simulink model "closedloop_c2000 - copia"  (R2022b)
settings: Solver=VariableStepAuto  StartTime=0.0  StopTime=10.0  RelTol=1e-3
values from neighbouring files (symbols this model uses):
  kaw = ki/kp    (= 100)    [closedloop_analysis - copia.m]
  ki = wc*R    (= 20)    [closedloop_analysis - copia.m]
  kp = wc*L    (= 0.2)    [closedloop_analysis - copia.m]
  PWMcounter_period = floor(fcpu/fsw)    [closedloop_analysis - copia.m]
  Ts = Tsw    (= 2.77777777778e-05)    [closedloop_analysis - copia.m]
  Vdc = 450    [closedloop_analysis - copia.m]
undefined symbols (not defined in the file or in its folder): ADCIN0, ADCIN1, ADCINA0, ADCINB0, bit, DCAEVT1, DCAEVT1FILT, Down, ended, Filtered, g_adc, input, of, offset, Single, Trip, TZ1, Up, version, Zone
libraries: c2802xlib x7, simulink x2, slpidlib x2

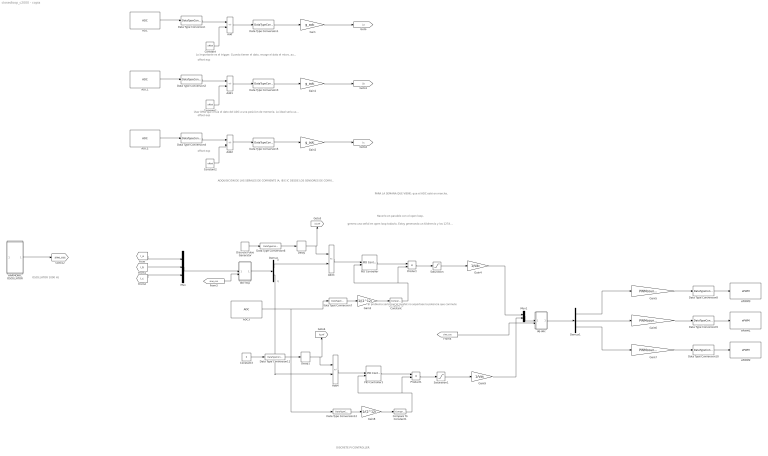
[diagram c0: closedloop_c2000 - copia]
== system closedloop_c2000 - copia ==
  note: PARA LA SEMANA QUE VIENE: que el ADC esté en marcha.
  note: El problema sería que el mosfet no soportase la potencia que conmute
  note: genero una señal en open loop todavía. Estoy generando un kilohercio y los 127A de pico. En teoría, el bucle cerrado tiene que estar midienddo esas dos partes de error, 0 prácticamente. Debería comportarse como el open loop. En el momento en el que cambias las consignas de bucle cerrado, el va a intentar modificar los PWMs porque le va a estar dando error. Ahí los PI se ponen en marchas y generan diferencias en las consignas de salida, y como la inyección siguie siendo del open loop, se van a saturar los PI porque por mucho que intenta el control llevar la señal, como las señales serán fijas, no hay modificación, el error se aculuma y se saturará.
  note: Hacerlo en paralelo con el open loop.
  note: Usar DMA que envia el dato del ADC a una posicion de memoria. Lo ideal seria usarlo. Avisa a un elemento y lo pone en posiciopn X. cuando lanza la interrupcion de procesado. Le podemos decir que solo avise al micro solo cuando los ADCs hayan terminado. Tenemos está opcion. Si no es grave el desfase, se puede dejar así, si vemos que necesitamos más precisión, mejor.
  note: Lo importante es el trigger. Cuando tienen el dato, recoge el dato el micro, aunque no sea en el mismo instante temporal, el tiempo de retardo debería ser despreciable.
  note: OSCILLATOR 1000 Hz
  note: DISCRETE PI CONTROLLER
  note: q
  note: d
  note: ADQUISICIÓN DE LAS SEÑALES DE CORRIENTE IA, IB E IC DESDE LOS SENSORES DE CORRIENTE HASTA EL MICRO A TRAVÉS DE LOS ADC
  note: offset exp
  note: offset exp
  note: offset exp
  ADC : c2802xlib/ADC  blkParamProc=C2000  ADCModule=1  samplingMode=Single sample mode  ADCResolution=12-bit (Single-ended input)  useSOC1=SOC0  useSOC2=SOC0_SOC1  SOCAcquisitionWindow=7  SOCTriggerSource=ePWM1_ADCSOCA  SOCInterruptTrigger=No ADCINT  Ts=Ts  dType=uint16  postInterrupt=off  interruptSel=ADCINT1  ADCINTContinuous=on  endma=off  chdma=1  conv1=ADCINA0  conv2=ADCINA0 and ADCINB0  conv1_Type4=ADCIN0  conv2_Type4=ADCIN0 and ADCIN1
  ADC1 : c2802xlib/ADC  blkParamProc=C2000  ADCModule=1  samplingMode=Single sample mode  ADCResolution=12-bit (Single-ended input)  useSOC1=SOC1  useSOC2=SOC0_SOC1  SOCAcquisitionWindow=7  SOCTriggerSource=ePWM1_ADCSOCA  SOCInterruptTrigger=No ADCINT  Ts=Ts  dType=uint16  postInterrupt=off  interruptSel=ADCINT1  ADCINTContinuous=off  endma=off  chdma=1  conv1=ADCINA1  conv2=ADCINA0 and ADCINB0  conv1_Type4=ADCIN0  conv2_Type4=ADCIN0 and ADCIN1
  ADC2 : c2802xlib/ADC  blkParamProc=C2000  ADCModule=1  samplingMode=Single sample mode  ADCResolution=12-bit (Single-ended input)  useSOC1=SOC3  useSOC2=SOC0_SOC1  SOCAcquisitionWindow=7  SOCTriggerSource=ePWM1_ADCSOCA  SOCInterruptTrigger=No ADCINT  Ts=Ts  dType=uint16  postInterrupt=off  interruptSel=ADCINT1  ADCINTContinuous=off  endma=off  chdma=1  conv1=ADCINA2  conv2=ADCINA0 and ADCINB0  conv1_Type4=ADCIN0  conv2_Type4=ADCIN0 and ADCIN1
  ADC3 : c2802xlib/ADC  blkParamProc=C2000  ADCModule=1  samplingMode=Single sample mode  ADCResolution=12-bit (Single-ended input)  useSOC1=SOC0  useSOC2=SOC0_SOC1  SOCAcquisitionWindow=7  SOCTriggerSource=Software  SOCInterruptTrigger=No ADCINT  Ts=0.0011  dType=uint16  postInterrupt=off  interruptSel=ADCINT1  ADCINTContinuous=off  endma=off  chdma=1  conv1=ADCINB3  conv2=ADCINA0 and ADCINB0  conv1_Type4=ADCIN0  conv2_Type4=ADCIN0 and ADCIN1
  Add{,1..4} (5 alike) : Sum  Inputs=+-
  Compare To Constant : simulink/Logic and Bit Operations/Compare To Constant  relop=>=  const=0.5  OutDataTypeStr=boolean
  Compare To Constant1 : simulink/Logic and Bit Operations/Compare To Constant  relop=>=  const=0.5  OutDataTypeStr=boolean
  Constant : Constant  Value=offset
  Constant1 : Constant  Value=offset
  Constant2 : Constant  Value=offset
  Constant3 : Constant  Value=0
  Data Type Conversion{,2,4,7..10,12} (8 alike) : DataTypeConversion  OutDataTypeStr=int16
  Data Type Conversion{1,3,5..6,11} (5 alike) : DataTypeConversion  OutDataTypeStr=single
  Delay : Delay  DelayLength=1  SampleTime=Ts/2
  Delay1 : Delay  DelayLength=1  SampleTime=Ts/2
  Demux : Demux  Outputs=2
  Demux1 : Demux  Outputs=3
  Discrete Pulse Generator : DiscretePulseGenerator  Amplitude=127  Period=120  PulseWidth=60  PhaseDelay=5  SampleTime=Ts
  Gain : Gain  Gain=g_adc
  Gain1 : Gain  Gain=g_adc
  Gain2 : Gain  Gain=g_adc
  Gain3 : Gain  Gain=1/(2^12)
  Gain4 : Gain  Gain=1/Vdc
  Gain5 : Gain  Gain=PWMcounter_period
  Gain6 : Gain  Gain=PWMcounter_period
  Gain7 : Gain  Gain=PWMcounter_period
  Gain8 : Gain  Gain=1/(2^12)
  Gain9 : Gain  Gain=1/Vdc
  HARMONIC OSCILLATOR : Subsystem
  Mux : Mux  Inputs=3
  Mux1 : Mux  Inputs=2
  PID Controller : slpidlib/PID Controller  Controller=PI  Form=Parallel  TimeDomain=Discrete-time  UseExternalTs=off  SampleTime=Ts  IntegratorMethod=Backward Euler  FilterMethod=Forward Euler  ControllerParametersSource=internal  P=kp  I=ki  UseKiTs=off  D=0  N=100  UseFilter=on  TunerSelectOption=Frequency Response Based  InitialConditionSource=internal  InitialConditionForIntegrator=0  InitialConditionForFilter=0  DifferentiatorICPrevScaledInput=0  ExternalReset=rising  TrackingMode=off  Kt=1  LimitOutput=on  SatLimitsSource=internal  UpperSaturationLimit=Vdc*0.98  LowerSaturationLimit=0  LinearizeAsGain=on  AntiWindupMode=back-calculation  Kb=kaw  LimitIntegrator=off  UpperIntegratorSaturationLimit=inf  LowerIntegratorSaturationLimit=-inf  POutMin=[]  POutMax=[]  IOutMin=[]  IOutMax=[]  DOutMin=[]  DOutMax=[]  NOutMin=[]  NOutMax=[]  SumOutMin=[]  SumOutMax=[]  SaturationOutMin=[]  SaturationOutMax=[]  PParamMin=[]  PParamMax=[]  IParamMin=[]  IParamMax=[]  DParamMin=[]  DParamMax=[]  NParamMin=[]  NParamMax=[]  KbParamMin=[]  KbParamMax=[]  KtParamMin=[]  KtParamMax=[]  KbOutMin=[]  KbOutMax=[]  KtOutMin=[]  KtOutMax=[]  IntegratorOutMin=[]  IntegratorOutMax=[]  FilterOutMin=[]  FilterOutMax=[]  SumI1OutMin=[]  SumI1OutMax=[]  SumI2OutMin=[]  SumI2OutMax=[]  SumI3OutMin=[]  SumI3OutMax=[]  SumI4OutMin=[]  SumI4OutMax=[]  SumDOutMin=[]  SumDOutMax=[]  DifferentiatorOutMin=[]  DifferentiatorOutMax=[]  FilterDiffOutCoefMin=[]  FilterDiffOutCoefMax=[]  ReciprocalOutMin=[]  ReciprocalOutMax=[]  SumDenOutMin=[]  SumDenOutMax=[]  SumNumOutMin=[]  SumNumOutMax=[]  DivideOutMin=[]  DivideOutMax=[]  UdiffTsProdOutMin=[]  UdiffTsProdOutMax=[]  NTsProdOutMin=[]  NTsProdOutMax=[]  UintegralTsProdOutMin=[]  UintegralTsProdOutMax=[]  UngainTsProdOutMin=[]  UngainTsProdOutMax=[]  ClampingZeroOutDataTypeStr=Inherit: Inherit via back propagation  ClampingZeroOutMin=[]  ClampingZeroOutMax=[]  FilterDenConstantOutDataTypeStr=Inherit: Inherit via back propagation  FilterDenConstantOutMin=[]  FilterDenConstantOutMax=[]  PCopyOutDataTypeStr=Inherit: Inherit via back propagation  PCopyOutMin=[]  PCopyOutMax=[]  NCopyOutDataTypeStr=Inherit: Inherit via back propagation  NCopyOutMin=[]  NCopyOutMax=[]  IntegratorContinuousStateAttributes=''  IntegratorStateMustResolveToSignalObject=off  IntegratorRTWStateStorageClass=Auto  FilterContinuousStateAttributes=''  FilterStateMustResolveToSignalObject=off  FilterRTWStateStorageClass=Auto  ParallelPVariant=InternalParameters  IdealPVariant=Disabled  IVariant=InternalParameters  DVariant=Disabled  IntegratorVariant=Discrete  SatVariant=Enabled  AWVariant=BackCalculation  PCopyVariant=Disabled  TRVariant=Disabled  FdbkBlocksVariant=Feedback  IdealPFdbkVariant=Passthrough  SatFdbkVariant=Enabled  DerivativeFilterVariant=Disabled  NVariant=Disabled  NCopyVariant=Disabled_SignalSpec  FilterICVariant=Disabled  IntegratorICVariant=InternalICs  ExternalResetVariant=ExternalReset  TRSumVariant=Passthrough  SumFdbkVariant=Enabled  SumVariant=Sum_PI  TsampFilterVariant=InternalTs  TsampNgainVariant=Passthrough  TsampIntegralVariant=Passthrough  ExternalSaturationOutDataTypeStr=Inherit: Same as second input
  PID Controller1 : slpidlib/PID Controller  Controller=PI  Form=Parallel  TimeDomain=Discrete-time  UseExternalTs=off  SampleTime=Ts  IntegratorMethod=Backward Euler  FilterMethod=Forward Euler  ControllerParametersSource=internal  P=kp  I=ki  UseKiTs=off  D=0  N=100  UseFilter=on  TunerSelectOption=Frequency Response Based  InitialConditionSource=internal  InitialConditionForIntegrator=0  InitialConditionForFilter=0  DifferentiatorICPrevScaledInput=0  ExternalReset=rising  TrackingMode=off  Kt=1  LimitOutput=on  SatLimitsSource=internal  UpperSaturationLimit=Vdc*0.98  LowerSaturationLimit=0  LinearizeAsGain=on  AntiWindupMode=back-calculation  Kb=kaw  LimitIntegrator=off  UpperIntegratorSaturationLimit=inf  LowerIntegratorSaturationLimit=-inf  POutMin=[]  POutMax=[]  IOutMin=[]  IOutMax=[]  DOutMin=[]  DOutMax=[]  NOutMin=[]  NOutMax=[]  SumOutMin=[]  SumOutMax=[]  SaturationOutMin=[]  SaturationOutMax=[]  PParamMin=[]  PParamMax=[]  IParamMin=[]  IParamMax=[]  DParamMin=[]  DParamMax=[]  NParamMin=[]  NParamMax=[]  KbParamMin=[]  KbParamMax=[]  KtParamMin=[]  KtParamMax=[]  KbOutMin=[]  KbOutMax=[]  KtOutMin=[]  KtOutMax=[]  IntegratorOutMin=[]  IntegratorOutMax=[]  FilterOutMin=[]  FilterOutMax=[]  SumI1OutMin=[]  SumI1OutMax=[]  SumI2OutMin=[]  SumI2OutMax=[]  SumI3OutMin=[]  SumI3OutMax=[]  SumI4OutMin=[]  SumI4OutMax=[]  SumDOutMin=[]  SumDOutMax=[]  DifferentiatorOutMin=[]  DifferentiatorOutMax=[]  FilterDiffOutCoefMin=[]  FilterDiffOutCoefMax=[]  ReciprocalOutMin=[]  ReciprocalOutMax=[]  SumDenOutMin=[]  SumDenOutMax=[]  SumNumOutMin=[]  SumNumOutMax=[]  DivideOutMin=[]  DivideOutMax=[]  UdiffTsProdOutMin=[]  UdiffTsProdOutMax=[]  NTsProdOutMin=[]  NTsProdOutMax=[]  UintegralTsProdOutMin=[]  UintegralTsProdOutMax=[]  UngainTsProdOutMin=[]  UngainTsProdOutMax=[]  ClampingZeroOutDataTypeStr=Inherit: Inherit via back propagation  ClampingZeroOutMin=[]  ClampingZeroOutMax=[]  FilterDenConstantOutDataTypeStr=Inherit: Inherit via back propagation  FilterDenConstantOutMin=[]  FilterDenConstantOutMax=[]  PCopyOutDataTypeStr=Inherit: Inherit via back propagation  PCopyOutMin=[]  PCopyOutMax=[]  NCopyOutDataTypeStr=Inherit: Inherit via back propagation  NCopyOutMin=[]  NCopyOutMax=[]  IntegratorContinuousStateAttributes=''  IntegratorStateMustResolveToSignalObject=off  IntegratorRTWStateStorageClass=Auto  FilterContinuousStateAttributes=''  FilterStateMustResolveToSignalObject=off  FilterRTWStateStorageClass=Auto  ParallelPVariant=InternalParameters  IdealPVariant=Disabled  IVariant=InternalParameters  DVariant=Disabled  IntegratorVariant=Discrete  SatVariant=Enabled  AWVariant=BackCalculation  PCopyVariant=Disabled  TRVariant=Disabled  FdbkBlocksVariant=Feedback  IdealPFdbkVariant=Passthrough  SatFdbkVariant=Enabled  DerivativeFilterVariant=Disabled  NVariant=Disabled  NCopyVariant=Disabled_SignalSpec  FilterICVariant=Disabled  IntegratorICVariant=InternalICs  ExternalResetVariant=ExternalReset  TRSumVariant=Passthrough  SumFdbkVariant=Enabled  SumVariant=Sum_PI  TsampFilterVariant=InternalTs  TsampNgainVariant=Passthrough  TsampIntegralVariant=Passthrough  ExternalSaturationOutDataTypeStr=Inherit: Same as second input
  Product : Product
  Product1 : Product
  Saturation : Saturate  UpperLimit=Vdc*0.98  LowerLimit=0
  Saturation1 : Saturate  UpperLimit=Vdc*0.98  LowerLimit=0
  abc-dq1 : Subsystem
  dq-abc : Subsystem
  ePWM1 : c2802xlib/ePWM  PwmType=C2000_Type4_F28002x  useModule=ePWM2  ePWMxLINKTBPRD=Not Linked  periodUnits=Clock cycles  timerSource=Specify via dialog  timerPeriod_clk=PWMcounter_period  timerPeriod_sec=50e-6  tbshadow=Counter equals to zero  countingMode=Up-Down  phaseActiveEnable=Disable  phaseDirection=Count down after sync  phaseActive=1111  synchronizationEnable=off  dcaevt1Sync=off  dcbevt1Sync=off  synchronizationOption=Disable  dcbevt1SyncOut=off  dcaevt1SyncOut=off  cmpdSyncOut=off  cmpcSyncOut=off  cmpbSyncOut=off  zeroSyncOut=on  swfSyncOut=off  perSynchronizationOption=Counter equals to period (CTR=PRD)  clockPrescale=1  HSclockPrescale=1  enswap=off  ePWMxAStatus=on  ePWMxAactionLogic1=Do nothing  ePWMxAactionLogic2=Do nothing  ePWMxAactionLogic3=Clear  ePWMxAactionLogic4=Set  ePWMxAactionLogic5=Do nothing  ePWMxAactionLogic6=Do nothing  ePWMxACSFenable=off  ePWMxACSFvalue=Forcing disable  ePWMxASFreload=Zero  ePWMxBStatus=off  ePWMxBactionLogic1=Set  ePWMxBactionLogic2=Do nothing  ePWMxBactionLogic3=Clear  ePWMxBactionLogic4=Set  ePWMxBactionLogic5=Do nothing  ePWMxBactionLogic6=Do nothing  ePWMxBCSFenable=off  ePWMxBCSFvalue=Forcing disable  ePWMxBSFreload=Zero  ePWNxBOutWay=on  ePWMxLINKCMPA=Not Linked  CMPAUnits=Clock cycles  CMPASource=Input port  CMPAValue_per=50  CMPAValue_clk=0  enCMPAshadow=Counter equals to zero (CTR=Zero)  ePWMxLINKCMPB=Not Linked  CMPBUnits=Clock cycles  CMPBSource=Specify via dialog  CMPBValue_per=50  CMPBValue_clk=0  enCMPBshadow=Counter equals to zero (CTR=Zero)  ePWMxLINKCMPC=Not Linked  CMPCUnits=Clock cycles  CMPCSource=Specify via dialog  CMPCValue_per=50  CMPCValue_clk=0  enCMPCshadow=Counter equals to zero (CTR=Zero)  ePWMxLINKCMPD=Not Linked  CMPDUnits=Clock cycles  CMPDSource=Specify via dialog  CMPDValue_per=50  CMPDValue_clk=32000  enCMPDshadow=Counter equals to zero (CTR=Zero)  enableDBePWMxA=on  enableDBePWMxB=on  enhalfcycle=off  DBpolarity=Active high complementary (AHC)  DBedgeDelay=Positive  DBSource_ePWMxA=ePWMxA  DBSource_ePWMxB=ePWMxA  DBPeriodUnits=Clock cycles  DBperiodSource=Specify via dialog  REDperiod=60  FEDperiod=60  REDperiod_sec=0  FEDperiod_sec=0  LoadModeDBRED=Immediate without using shadow  LoadModeDBFED=Immediate without using shadow  adcstartModuleA=on  adcrequestEventA=First event  adcstartEventA=Counter equals to zero (CTR=Zero)  adcstartEventA_type2=Counter equals to zero (CTR=Zero)  adcstartModuleB=off  adcrequestEventB=First event  adcstartEventB=Counter equals to zero (CTR=Zero)  adcstartEventB_type2=Counter equals to zero (CTR=Zero)  intEn=off  intPrd=First event  intSel=Counter equals to zero (CTR=Zero)  intSel_type2=Counter equals to zero (CTR=Zero)  hrpe=off  enHRPWM=off  HRPWM_LoadMode=Counter equals to period (CTR=PRD)  HRPWM_CTLMode=Duty or Period control mode  HRPWM_EDGMode=Both edge  hrpeb=off  enHRPWMB=off  HRPWM_LoadModeB=Counter equals to zero (CTR=ZERO)  HRPWM_CTLModeB=Duty or Period control mode  HRPWM_EDGModeB=Both edge  enHRDBRED=off  enHRDBFED=off  enSFO=on  enautoconv=on  chopperEnable=off  chopperFrequency=1  chopperFirstwidth=1  chopperDuty=12.5%  tripZonesource=Specify via dialog  tzselOSHT1=off  tzselOSHT2=off  tzselOSHT3=off  tzselOSHDCAEV1=off  tzselOSHDCBEV1=off  tzselCBC1=on  tzselCBC2=off  tzselCBC3=off  tzselCBCDCAEV2=off  tzselCBCDCBEV2=off  tzselOSHT4=off  tzselOSHT5=off  tzselOSHT6=off  tzselCBC4=off  tzselCBC5=off  tzselCBC6=off  enTzOstIntr=off  enTzCbcIntr=on  enTzDCAEVT1Intr=off  enTzDCAEVT2Intr=off  enTzDCBEVT1Intr=off  enTzDCBEVT2Intr=off  ePWMxAforced=Low  ePWMxBforced=Low  DCAEVT1forced=No action  DCBEVT1forced=No action  DCAEVT2forced=No action  DCBEVT2forced=No action  dcah=Trip Zone 1 input (TZ1)  dcal=Trip Zone 1 input (TZ1)  dcbh=Trip Zone 1 input (TZ1)  dcbl=Trip Zone 1 input (TZ1)  dcah_type2=GPTRIP5SEL  dcal_type2=GPTRIP5SEL  dcbh_type2=GPTRIP8SEL  dcbl_type2=GPTRIP7SEL  gendcaevt1=DCAH=high and DCAL=don't care  gendcaevt2=Event disabled  gendcbevt1=Event disabled  gendcbevt2=Event disabled  dcaevt1src=DCAEVT1 with sync  dcaevt2src=DCAEVT2 with sync  dcbevt1src=DCBEVT1 with sync  dcbevt2src=DCBEVT2 with sync  pulsesel=Counter equals to zero (CTR=Zero)  blankinv=off  blankoffset=0  blankwidth=0  evsrcsel=Filtered version of DCAEVT1 (DCAEVT1FILT)  encape=off
  ePWM2 : c2802xlib/ePWM  PwmType=C2000_Type4_F28002x  useModule=ePWM3  ePWMxLINKTBPRD=Not Linked  periodUnits=Clock cycles  timerSource=Specify via dialog  timerPeriod_clk=PWMcounter_period  timerPeriod_sec=50e-6  tbshadow=Counter equals to zero  countingMode=Up-Down  phaseActiveEnable=Disable  phaseDirection=Count down after sync  phaseActive=1111  synchronizationEnable=off  dcaevt1Sync=off  dcbevt1Sync=off  synchronizationOption=Disable  dcbevt1SyncOut=off  dcaevt1SyncOut=off  cmpdSyncOut=off  cmpcSyncOut=off  cmpbSyncOut=off  zeroSyncOut=on  swfSyncOut=off  perSynchronizationOption=Counter equals to period (CTR=PRD)  clockPrescale=1  HSclockPrescale=1  enswap=off  ePWMxAStatus=on  ePWMxAactionLogic1=Do nothing  ePWMxAactionLogic2=Do nothing  ePWMxAactionLogic3=Clear  ePWMxAactionLogic4=Set  ePWMxAactionLogic5=Do nothing  ePWMxAactionLogic6=Do nothing  ePWMxACSFenable=off  ePWMxACSFvalue=Forcing disable  ePWMxASFreload=Zero  ePWMxBStatus=off  ePWMxBactionLogic1=Set  ePWMxBactionLogic2=Do nothing  ePWMxBactionLogic3=Clear  ePWMxBactionLogic4=Set  ePWMxBactionLogic5=Do nothing  ePWMxBactionLogic6=Do nothing  ePWMxBCSFenable=off  ePWMxBCSFvalue=Forcing disable  ePWMxBSFreload=Zero  ePWNxBOutWay=on  ePWMxLINKCMPA=Not Linked  CMPAUnits=Clock cycles  CMPASource=Input port  CMPAValue_per=50  CMPAValue_clk=0  enCMPAshadow=Counter equals to zero (CTR=Zero)  ePWMxLINKCMPB=Not Linked  CMPBUnits=Clock cycles  CMPBSource=Specify via dialog  CMPBValue_per=50  CMPBValue_clk=0  enCMPBshadow=Counter equals to zero (CTR=Zero)  ePWMxLINKCMPC=Not Linked  CMPCUnits=Clock cycles  CMPCSource=Specify via dialog  CMPCValue_per=50  CMPCValue_clk=0  enCMPCshadow=Counter equals to zero (CTR=Zero)  ePWMxLINKCMPD=Not Linked  CMPDUnits=Clock cycles  CMPDSource=Specify via dialog  CMPDValue_per=50  CMPDValue_clk=32000  enCMPDshadow=Counter equals to zero (CTR=Zero)  enableDBePWMxA=on  enableDBePWMxB=on  enhalfcycle=off  DBpolarity=Active high complementary (AHC)  DBedgeDelay=Positive  DBSource_ePWMxA=ePWMxA  DBSource_ePWMxB=ePWMxA  DBPeriodUnits=Clock cycles  DBperiodSource=Specify via dialog  REDperiod=60  FEDperiod=60  REDperiod_sec=0  FEDperiod_sec=0  LoadModeDBRED=Immediate without using shadow  LoadModeDBFED=Immediate without using shadow  adcstartModuleA=on  adcrequestEventA=First event  adcstartEventA=Counter equals to zero (CTR=Zero)  adcstartEventA_type2=Counter equals to zero (CTR=Zero)  adcstartModuleB=off  adcrequestEventB=First event  adcstartEventB=Counter equals to zero (CTR=Zero)  adcstartEventB_type2=Counter equals to zero (CTR=Zero)  intEn=off  intPrd=First event  intSel=Counter equals to zero (CTR=Zero)  intSel_type2=Counter equals to zero (CTR=Zero)  hrpe=off  enHRPWM=off  HRPWM_LoadMode=Counter equals to period (CTR=PRD)  HRPWM_CTLMode=Duty or Period control mode  HRPWM_EDGMode=Both edge  hrpeb=off  enHRPWMB=off  HRPWM_LoadModeB=Counter equals to zero (CTR=ZERO)  HRPWM_CTLModeB=Duty or Period control mode  HRPWM_EDGModeB=Both edge  enHRDBRED=off  enHRDBFED=off  enSFO=on  enautoconv=on  chopperEnable=off  chopperFrequency=1  chopperFirstwidth=1  chopperDuty=12.5%  tripZonesource=Specify via dialog  tzselOSHT1=off  tzselOSHT2=off  tzselOSHT3=off  tzselOSHDCAEV1=off  tzselOSHDCBEV1=off  tzselCBC1=on  tzselCBC2=off  tzselCBC3=off  tzselCBCDCAEV2=off  tzselCBCDCBEV2=off  tzselOSHT4=off  tzselOSHT5=off  tzselOSHT6=off  tzselCBC4=off  tzselCBC5=off  tzselCBC6=off  enTzOstIntr=off  enTzCbcIntr=on  enTzDCAEVT1Intr=off  enTzDCAEVT2Intr=off  enTzDCBEVT1Intr=off  enTzDCBEVT2Intr=off  ePWMxAforced=Low  ePWMxBforced=Low  DCAEVT1forced=No action  DCBEVT1forced=No action  DCAEVT2forced=No action  DCBEVT2forced=No action  dcah=Trip Zone 1 input (TZ1)  dcal=Trip Zone 1 input (TZ1)  dcbh=Trip Zone 1 input (TZ1)  dcbl=Trip Zone 1 input (TZ1)  dcah_type2=GPTRIP5SEL  dcal_type2=GPTRIP5SEL  dcbh_type2=GPTRIP8SEL  dcbl_type2=GPTRIP7SEL  gendcaevt1=DCAH=high and DCAL=don't care  gendcaevt2=Event disabled  gendcbevt1=Event disabled  gendcbevt2=Event disabled  dcaevt1src=DCAEVT1 with sync  dcaevt2src=DCAEVT2 with sync  dcbevt1src=DCBEVT1 with sync  dcbevt2src=DCBEVT2 with sync  pulsesel=Counter equals to zero (CTR=Zero)  blankinv=off  blankoffset=0  blankwidth=0  evsrcsel=Filtered version of DCAEVT1 (DCAEVT1FILT)  encape=off
  ePWM3 : c2802xlib/ePWM  PwmType=C2000_Type4_F28002x  useModule=ePWM1  ePWMxLINKTBPRD=Not Linked  periodUnits=Clock cycles  timerSource=Specify via dialog  timerPeriod_clk=PWMcounter_period  timerPeriod_sec=50e-6  tbshadow=Counter equals to zero  countingMode=Up-Down  phaseActiveEnable=Disable  phaseDirection=Count down after sync  phaseActive=1111  synchronizationEnable=off  dcaevt1Sync=off  dcbevt1Sync=off  synchronizationOption=Disable  dcbevt1SyncOut=off  dcaevt1SyncOut=off  cmpdSyncOut=off  cmpcSyncOut=off  cmpbSyncOut=off  zeroSyncOut=on  swfSyncOut=off  perSynchronizationOption=Counter equals to period (CTR=PRD)  clockPrescale=1  HSclockPrescale=1  enswap=off  ePWMxAStatus=on  ePWMxAactionLogic1=Do nothing  ePWMxAactionLogic2=Do nothing  ePWMxAactionLogic3=Clear  ePWMxAactionLogic4=Set  ePWMxAactionLogic5=Do nothing  ePWMxAactionLogic6=Do nothing  ePWMxACSFenable=off  ePWMxACSFvalue=Forcing disable  ePWMxASFreload=Zero  ePWMxBStatus=off  ePWMxBactionLogic1=Set  ePWMxBactionLogic2=Do nothing  ePWMxBactionLogic3=Clear  ePWMxBactionLogic4=Set  ePWMxBactionLogic5=Do nothing  ePWMxBactionLogic6=Do nothing  ePWMxBCSFenable=off  ePWMxBCSFvalue=Forcing disable  ePWMxBSFreload=Zero  ePWNxBOutWay=on  ePWMxLINKCMPA=Not Linked  CMPAUnits=Clock cycles  CMPASource=Input port  CMPAValue_per=50  CMPAValue_clk=0  enCMPAshadow=Counter equals to zero (CTR=Zero)  ePWMxLINKCMPB=Not Linked  CMPBUnits=Clock cycles  CMPBSource=Specify via dialog  CMPBValue_per=50  CMPBValue_clk=0  enCMPBshadow=Counter equals to zero (CTR=Zero)  ePWMxLINKCMPC=Not Linked  CMPCUnits=Clock cycles  CMPCSource=Specify via dialog  CMPCValue_per=50  CMPCValue_clk=0  enCMPCshadow=Counter equals to zero (CTR=Zero)  ePWMxLINKCMPD=Not Linked  CMPDUnits=Clock cycles  CMPDSource=Specify via dialog  CMPDValue_per=50  CMPDValue_clk=32000  enCMPDshadow=Counter equals to zero (CTR=Zero)  enableDBePWMxA=on  enableDBePWMxB=on  enhalfcycle=off  DBpolarity=Active high complementary (AHC)  DBedgeDelay=Positive  DBSource_ePWMxA=ePWMxA  DBSource_ePWMxB=ePWMxA  DBPeriodUnits=Clock cycles  DBperiodSource=Specify via dialog  REDperiod=60  FEDperiod=60  REDperiod_sec=0  FEDperiod_sec=0  LoadModeDBRED=Immediate without using shadow  LoadModeDBFED=Immediate without using shadow  adcstartModuleA=on  adcrequestEventA=First event  adcstartEventA=Counter equals to zero (CTR=Zero)  adcstartEventA_type2=Counter equals to zero (CTR=Zero)  adcstartModuleB=off  adcrequestEventB=First event  adcstartEventB=Counter equals to zero (CTR=Zero)  adcstartEventB_type2=Counter equals to zero (CTR=Zero)  intEn=off  intPrd=First event  intSel=Counter equals to zero (CTR=Zero)  intSel_type2=Counter equals to zero (CTR=Zero)  hrpe=off  enHRPWM=off  HRPWM_LoadMode=Counter equals to period (CTR=PRD)  HRPWM_CTLMode=Duty or Period control mode  HRPWM_EDGMode=Both edge  hrpeb=off  enHRPWMB=off  HRPWM_LoadModeB=Counter equals to zero (CTR=ZERO)  HRPWM_CTLModeB=Duty or Period control mode  HRPWM_EDGModeB=Both edge  enHRDBRED=off  enHRDBFED=off  enSFO=on  enautoconv=on  chopperEnable=off  chopperFrequency=1  chopperFirstwidth=1  chopperDuty=12.5%  tripZonesource=Specify via dialog  tzselOSHT1=off  tzselOSHT2=off  tzselOSHT3=off  tzselOSHDCAEV1=off  tzselOSHDCBEV1=off  tzselCBC1=on  tzselCBC2=off  tzselCBC3=off  tzselCBCDCAEV2=off  tzselCBCDCBEV2=off  tzselOSHT4=off  tzselOSHT5=off  tzselOSHT6=off  tzselCBC4=off  tzselCBC5=off  tzselCBC6=off  enTzOstIntr=off  enTzCbcIntr=on  enTzDCAEVT1Intr=off  enTzDCAEVT2Intr=off  enTzDCBEVT1Intr=off  enTzDCBEVT2Intr=off  ePWMxAforced=Low  ePWMxBforced=Low  DCAEVT1forced=No action  DCBEVT1forced=No action  DCAEVT2forced=No action  DCBEVT2forced=No action  dcah=Trip Zone 1 input (TZ1)  dcal=Trip Zone 1 input (TZ1)  dcbh=Trip Zone 1 input (TZ1)  dcbl=Trip Zone 1 input (TZ1)  dcah_type2=GPTRIP5SEL  dcal_type2=GPTRIP5SEL  dcbh_type2=GPTRIP8SEL  dcbl_type2=GPTRIP7SEL  gendcaevt1=DCAH=high and DCAL=don't care  gendcaevt2=Event disabled  gendcbevt1=Event disabled  gendcbevt2=Event disabled  dcaevt1src=DCAEVT1 with sync  dcaevt2src=DCAEVT2 with sync  dcbevt1src=DCBEVT1 with sync  dcbevt2src=DCBEVT2 with sync  pulsesel=Counter equals to zero (CTR=Zero)  blankinv=off  blankoffset=0  blankwidth=0  evsrcsel=Filtered version of DCAEVT1 (DCAEVT1FILT)  encape=off
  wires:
  ADC/1 -> Data Type Conversion/1
  Data Type Conversion/1 -> Add/1
  Constant/1 -> Add/2
  Add/1 -> Data Type Conversion1/1
  Data Type Conversion1/1 -> Gain/1
  Gain/1 -> [i_a]
  Gain1/1 -> [i_b]
  Data Type Conversion3/1 -> Gain1/1
  Add1/1 -> Data Type Conversion3/1
  Data Type Conversion2/1 -> Add1/1
  ADC1/1 -> Data Type Conversion2/1
  Constant1/1 -> Add1/2
  Gain2/1 -> [i_c]
  Data Type Conversion5/1 -> Gain2/1
  Add2/1 -> Data Type Conversion5/1
  Data Type Conversion4/1 -> Add2/1
  ADC2/1 -> Data Type Conversion4/1
  Constant2/1 -> Add2/2
  [i_a] -> Mux/1
  [i_b] -> Mux/2
  [i_c] -> Mux/3
  Mux/1 -> abc-dq1/1(abc)
  HARMONIC OSCILLATOR/1(sin-cos) -> [sine_cos]
  [sine_cos] -> abc-dq1/2(sin-cos)
  abc-dq1/1(dq) -> Demux/1
  Discrete Pulse Generator/1 -> Data Type Conversion6/1
  Data Type Conversion6/1 -> Delay/1
  Demux/1 -> Add3/2
  Delay/1 -> Add3/1, [id_ref]
  Add3/1 -> PID Controller/1
  Data Type Conversion7/1 -> Gain3/1
  Gain3/1 -> Compare To Constant/1
  Compare To Constant/1 -> Product/2, PID Controller/2
  PID Controller/1 -> Product/1
  Product/1 -> Saturation/1
  Saturation/1 -> Gain4/1
  [sine_cos] -> dq-abc/2(sin-cos)
  dq-abc/1(abc) -> Demux1/1
  Demux1/1 -> Gain5/1
  Demux1/2 -> Gain6/1
  Demux1/3 -> Gain7/1
  Data Type Conversion8/1 -> ePWM3/1
  Gain5/1 -> Data Type Conversion8/1
  Data Type Conversion9/1 -> ePWM1/1
  Gain6/1 -> Data Type Conversion9/1
  Data Type Conversion10/1 -> ePWM2/1
  Gain7/1 -> Data Type Conversion10/1
  Data Type Conversion12/1 -> Gain8/1
  Add4/1 -> PID Controller1/1
  Compare To Constant1/1 -> Product1/2, PID Controller1/2
  Product1/1 -> Saturation1/1
  Demux/2 -> Add4/2
  Delay1/1 -> Add4/1, [iq_ref]
  ADC3/1 -> Data Type Conversion7/1, Data Type Conversion12/1
  Saturation1/1 -> Gain9/1
  Gain8/1 -> Compare To Constant1/1
  PID Controller1/1 -> Product1/1
  Data Type Conversion11/1 -> Delay1/1
  Constant3/1 -> Data Type Conversion11/1
  Mux1/1 -> dq-abc/1(dq)
  Gain4/1 -> Mux1/1
  Gain9/1 -> Mux1/2

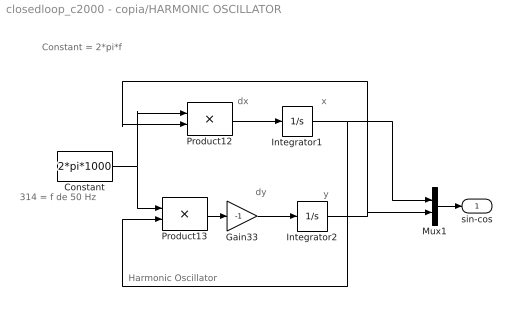
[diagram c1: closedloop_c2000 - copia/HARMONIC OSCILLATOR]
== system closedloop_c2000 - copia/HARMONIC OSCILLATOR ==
  note: 314 = f de 50 Hz
  note: Constant = 2*pi*f
  note: Harmonic Oscillator
  note: dy
  note: dx
  note: y
  note: x
  Constant : Constant  Value=2*pi*1000
  Gain33 : Gain  Gain=-1  SaturateOnIntegerOverflow=on
  Integrator1 : Integrator  InitialCondition=1  LimitOutput=on  UpperSaturationLimit=1  LowerSaturationLimit=-1
  Integrator2 : Integrator  LimitOutput=on  UpperSaturationLimit=1  LowerSaturationLimit=-1
  Mux1 : Mux  Inputs=2
  Product12 : Product  SaturateOnIntegerOverflow=on
  Product13 : Product  SaturateOnIntegerOverflow=on
  sin-cos : Outport  VectorParamsAs1DForOutWhenUnconnected=off
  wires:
  Constant/1 -> Product13/1, Product12/1
  Gain33/1 -> Integrator2/1
  Product12/1 -> Integrator1/1
  Product13/1 -> Gain33/1
  Integrator1/1 -> Product13/2, Mux1/1
  Integrator2/1 -> Product12/2, Mux1/2
  Mux1/1 -> sin-cos/1

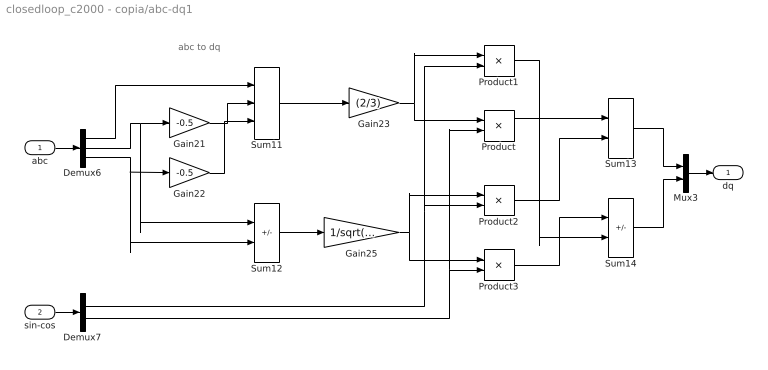
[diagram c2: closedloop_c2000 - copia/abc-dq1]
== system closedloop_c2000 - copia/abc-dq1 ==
  note: abc to dq
  abc : Inport
  sin-cos : Inport  Port=2
  Demux6 : Demux  Outputs=3
  Demux7 : Demux  Outputs=2
  Gain21 : Gain  Gain=-0.5
  Gain22 : Gain  Gain=-0.5
  Gain23 : Gain  Gain=(2/3)
  Gain25 : Gain  Gain=1/sqrt(3)
  Mux3 : Mux  Inputs=2
  Product{,1..3} (4 alike) : Product  RndMeth=Zero
  Sum11 : Sum  Inputs=|+++
  Sum12 : Sum  Inputs=|+-
  Sum13 : Sum  Inputs=|++
  Sum14 : Sum  Inputs=|+-
  dq : Outport  VectorParamsAs1DForOutWhenUnconnected=off
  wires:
  Sum11/1 -> Gain23/1
  Sum12/1 -> Gain25/1
  Demux6/3 -> Gain22/1, Sum12/2
  Demux6/2 -> Gain21/1, Sum12/1
  Demux6/1 -> Sum11/1
  Gain21/1 -> Sum11/2
  Gain22/1 -> Sum11/3
  Gain23/1 -> Product/1, Product1/1
  Demux7/2 -> Product/2, Product3/2
  Demux7/1 -> Product1/2, Product2/2
  Gain25/1 -> Product2/1, Product3/1
  Product/1 -> Sum13/1
  Product2/1 -> Sum13/2
  Product3/1 -> Sum14/1
  Product1/1 -> Sum14/2
  Sum13/1 -> Mux3/1
  Sum14/1 -> Mux3/2
  abc/1 -> Demux6/1
  Mux3/1 -> dq/1
  sin-cos/1 -> Demux7/1

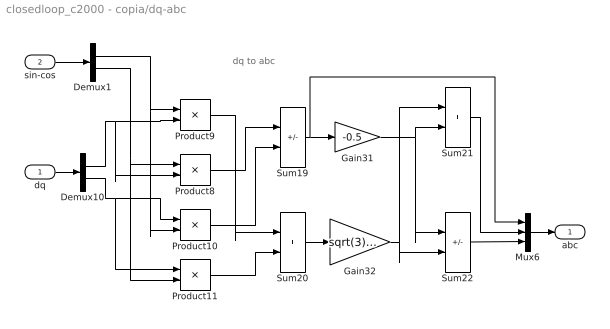
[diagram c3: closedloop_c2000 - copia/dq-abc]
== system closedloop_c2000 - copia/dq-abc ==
  note: dq to abc
  dq : Inport
  sin-cos : Inport  Port=2
  Demux1 : Demux  Outputs=2
  Demux10 : Demux  Outputs=2
  Gain31 : Gain  Gain=-0.5
  Gain32 : Gain  Gain=sqrt(3)/2
  Mux6 : Mux  Inputs=3
  Product{8..11} (4 alike) : Product  RndMeth=Zero
  Sum19 : Sum  Inputs=|+-
  Sum20 : Sum  Inputs=|++
  Sum21 : Sum  Inputs=|++
  Sum22 : Sum  Inputs=|+-
  abc : Outport  VectorParamsAs1DForOutWhenUnconnected=off
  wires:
  Sum22/1 -> Mux6/3
  Sum21/1 -> Mux6/2
  Demux10/2 -> Product10/1, Product11/1
  Demux10/1 -> Product9/2, Product8/2
  Gain31/1 -> Sum21/2, Sum22/1
  Gain32/1 -> Sum21/1, Sum22/2
  Sum19/1 -> Gain31/1, Mux6/1
  Sum20/1 -> Gain32/1
  Product10/1 -> Sum19/2
  Product11/1 -> Sum20/2
  Product9/1 -> Sum20/1
  Product8/1 -> Sum19/1
  Demux1/1 -> Product10/2, Product9/1
  Demux1/2 -> Product11/2, Product8/1
  dq/1 -> Demux10/1
  Mux6/1 -> abc/1
  sin-cos/1 -> Demux1/1
